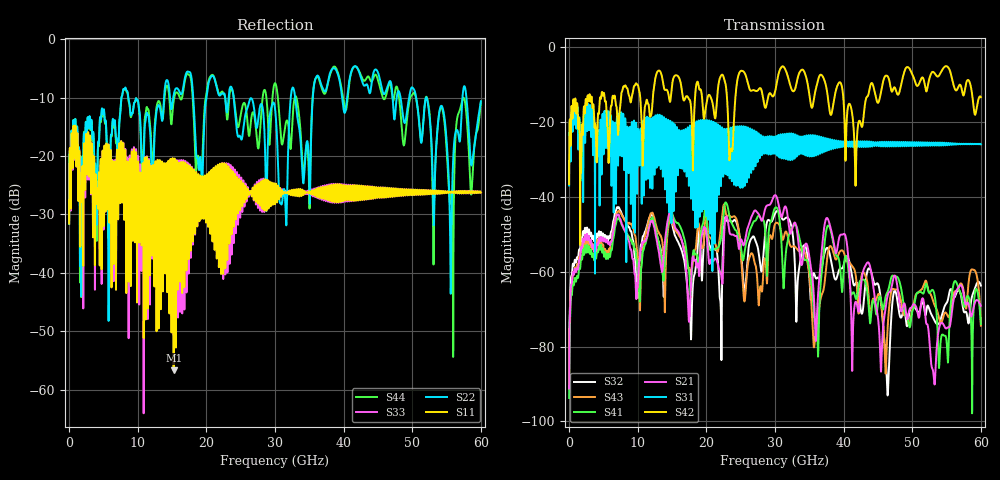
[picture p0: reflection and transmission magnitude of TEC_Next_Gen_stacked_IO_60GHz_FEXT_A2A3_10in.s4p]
!! CHANNEL DESCRIPTION:  Next Generation 28Gbps Press-fit Stacked I/O Connector
!!  with 10" 5-6-5 Megtron 6 Stripline trace on host side and 1.25" 7-5-7 Megtron 6 Microstrip trace on plug side
!! HOST PCB DESCRIPTION:  PCB thickness 3.425 mm
!!  26 Layer Board, 15 GND planes, 4 Layer route-out on Layers 7,11,17,21, 8mil stub on vias
!!  Pairs on following layers
!!  Layer 07 - A02A03 A14A15 D05D06
!!  Layer 11 - D020D3 C05C06 D14D15
!!  Layer 17 - C02C03 B05B06 C14C15
!!  Layer 21 - B02B03 A05A06 B14B15
!! CONNECTOR DESCRIPTION:  Next Generation 28Gbps Press-fit Stacked I/O Connector
!! PLUG-IN CARD DESCRIPTION:  PCB thickness 1mm thick
!!  6 Layer Board, 4 GND planes, 0.35 x 1.4mm mating pads
!!  Micro-strip diff traces referenced to GND plane 3mils down, 2nd GND plane 17mils from top of board
!!  PCB GND planes are symmetric
!! MODEL DESCRIPTION: TE Connectivity S-parameter model produced from Macro-model, Extracted .s4p FEXT (Victim B05B06 - Aggressor A02A03)
!! MODEL DATE: 5/15/2014 CR32f, FPR23
!! MODEL STATUS: Developmental
!! MODEL GEOMETRY: 4 Rows - Rows A, B, C, D. 3 pairs in each row, 12 total pairs
!! MODEL FREQUENCY RANGE: DC to 60 GHz in 10 MHz frequency steps
!! MODEL EDGE RATE LIMITATION: 8.33 ps (Using conservative 0.5/Fmax rule of thumb)
!! TIME-DOMAIN TRANSFORM CAUTIONS:
!! 1.) Do not simulate transient edge rates faster than the number listed above.  Edge
!!  rates faster than this number contain significant spectral content at frequencies
!!  above the model's highest frequency.
!! 2.) Even when simulating edge rates that are slower than the number listed above, be
!!  aware that the best time resolution possible with a direct iFFT is (1 / 2Fmax).
!!  As a result, time resolution is typically not adequate for most time-domain
!!  simulations unless tricks such as frequency-domain zero-padding and windowing are
!!  used to minimize leakage and aliasing.
!! 3.) Because the model has a uniform frequency step, a direct iFFT will result in an
!!  impulse that that has a time length given by either (1 / Fstep) or (1 / 2Fstep),
!!  depending on the transform being used.  Care has been taken in selecting the
!!  frequency step to ensure a settled impulse response for the model.  Therefore,
!!  convolution with the model's impulse response should present no issues.  However,
!!  if directly concatenating s-parameter models in the frequency domain a user must
!!  either interpolate necessary interim frequencies or complete impulse response
!!  zero-padding.  Impulse response zero-padding is more difficult, but more accurate.
!! PORT DEFINITIONS:
!! Port  1  ----->  Host A02		B05 Module <-----  Port  2
!! Port  3  ----->  Host A03		B06 Module <-----  Port  4
! Touchstone data
! Created: 29-Sep-2014 by IdEM R2011 (7.0.3)
# Hz S MA R 50
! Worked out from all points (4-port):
!   6000 points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, 10 MHz to 60 GHz, reference 50 ohm
!   strongest paths, dB at 10 MHz, 15.01 GHz, 30.01 GHz, 45.01 GHz, 60 GHz:
!     S42: -36.6, -10.1, -12.0, -14.9, -13.4
!     S31: -37.0, -21.6, -28.4, -25.5, -26.0
!     S21: -91.2, -44.9, -39.6, -72.4, -69.1
!     S41: -93.7, -44.3, -43.0, -68.4, -74.0
!     S43: -91.3, -46.5, -47.3, -66.1, -74.4
!     S32: -89.1, -47.2, -44.5, -63.3, -63.7
!   lowest |S11| = -56.6 dB at 15.24 GHz (marker M1), VSWR 1.00, Z = 50 - j0.145 ohm
!   |S11| at or under -10 dB: start of sweep to end of sweep
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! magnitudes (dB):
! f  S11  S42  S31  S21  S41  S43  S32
! 10 MHz  -31.5  -36.6  -37.0  -91.2  -93.7  -91.3  -89.1
! 2.33 GHz  -24.4  -16.9  -25.1  -50.1  -53.0  -51.0  -48.3
! 15.24 GHz  -56.6  -8.1  -36.2  -46.7  -45.6  -47.8  -49.0
! 17.47 GHz  -27.6  -13.9  -35.5  -73.3  -59.7  -59.0  -67.7
! 30.41 GHz  -25.3  -8.1  -26.1  -41.0  -43.5  -47.0  -43.7
! 46.31 GHz  -25.7  -7.6  -26.0  -67.3  -65.7  -78.8  -89.5
! 60 GHz  -26.3  -13.4  -26.0  -69.1  -74.0  -74.4  -63.7
